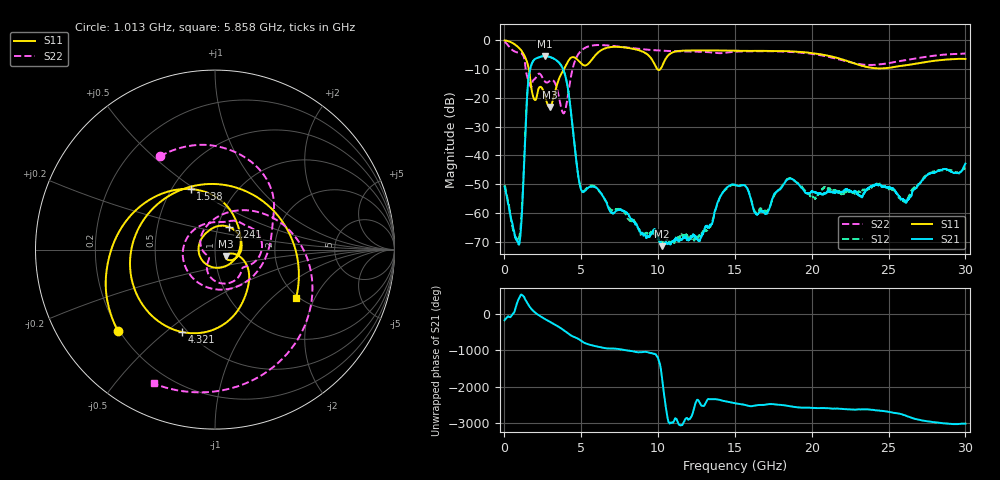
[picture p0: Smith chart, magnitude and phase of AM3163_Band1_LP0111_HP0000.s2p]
!Agilent Technologies,E8364B,MY43040894,A.07.50.67
!Agilent E8364B: A.07.50.67
!Date: Thursday, August 20, 2020 11:25:39
!Correction: S11(Full 2 Port(1,2))
!S21(Full 2 Port(1,2))
!S12(Full 2 Port(1,2))
!S22(Full 2 Port(1,2))
!S2P File: Measurements: S11, S21, S12, S22:
# Hz S  dB  R 50
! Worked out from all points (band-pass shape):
!   3201 points, 10 MHz to 30 GHz, reference 50 ohm
!   highest |S21| = -5.49 dB at 2.615 GHz (marker M1); lowest = -71.5 dB at 10.26 GHz (marker M2)
!   |S21| within 3 dB of the highest: 1.755 GHz to 3.66 GHz (1.905 GHz wide, 70.3 % of centre)
!   lowest |S11| = -23.2 dB at 2.934 GHz (marker M3), VSWR 1.15, Z = 56.2 - j3.94 ohm
!   |S11| at or under -10 dB: 1.588 GHz to 3.878 GHz (2.289 GHz wide, 83.8 % of centre); 9.942 GHz to 10.15 GHz (209.5 MHz wide, 2.08 % of centre)
!   |S22| runs from -25.4 to -0.5 dB; largest |S21 - S12| = 0.0054
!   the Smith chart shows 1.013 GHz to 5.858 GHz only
!   S11 on the Smith chart (normalised r, x): 1.013 GHz: 0.19, -0.35; 1.538 GHz: 0.62, +0.48; 2.241 GHz: 1.13, +0.29; 4.321 GHz: 0.47, -0.57; 5.858 GHz: 1.94, -1.44
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1e7  -0.07 -8.8  -50.87 -167.7  -50.17 -80.1  -0.53 -23.3
5.441969e8  -1.00 -72.5  -64.25 2.8  -65.37 120.7  -3.52 -150.0
1.012791e9  -3.02 -140.1  -69.09 120.7  -66.76 -5.9  -4.38 120.5
1.537616e9  -8.79 111.9  -14.92 -93.1  -14.90 -93.2  -13.68 -116.1
1.903119e9  -20.09 -99.0  -6.96 73.8  -6.96 73.7  -13.73 47.2
2.240506e9  -16.57 58.5  -5.95 -36.2  -5.95 -36.3  -11.59 10.9
2.615381e9  -18.99 -30.7  -5.49 -133.4  -5.50 -133.5  -14.22 -28.9
2.934025e9  -23.18 -30.1  -5.76 150.6  -5.77 150.5  -14.19 -43.4
3.496338e9  -14.21 -25.6  -7.47 15.9  -7.49 16.0  -18.57 -112.4
4.321062e9  -6.11 -112.0  -24.59 132.9  -24.55 133.0  -12.84 67.8
5.014581e9  -8.19 126.5  -52.19 -23.1  -51.87 -24.2  -3.52 -43.4
5.85805e9  -5.58 -30.8  -50.94 -157.2  -50.68 -156.2  -1.72 -114.7
6.542197e9  -2.83 -103.4  -55.23 143.1  -55.38 145.8  -1.72 -155.6
7.5075e9  -2.33 -169.9  -58.66 113.6  -58.59 112.0  -2.22 158.2
1.000979e10  -10.30 86.3  -68.52 -147.4  -69.12 133.5  -3.54 60.0
1.026283e10  -8.99 99.9  -71.52 26.0  -69.82 -80.1  -3.63 50.9
1.241836e10  -3.54 6.7  -68.15 55.4  -68.92 174.6  -3.96 -22.4
1.5005e10  -3.63 -72.3  -50.21 67.1  -50.32 68.6  -3.96 -90.6
2.000958e10  -4.44 163.2  -52.37 -55.8  -54.58 -49.8  -4.71 136.2
2.275554e10  -8.03 59.8  -52.68 -106.0  -52.80 -102.0  -7.97 20.8
2.500479e10  -9.59 -62.1  -51.17 -165.2  -51.57 -165.4  -7.97 -92.5
3e10  -6.50 104.2  -42.85 -133.8  -44.33 -129.3  -4.62 101.7
